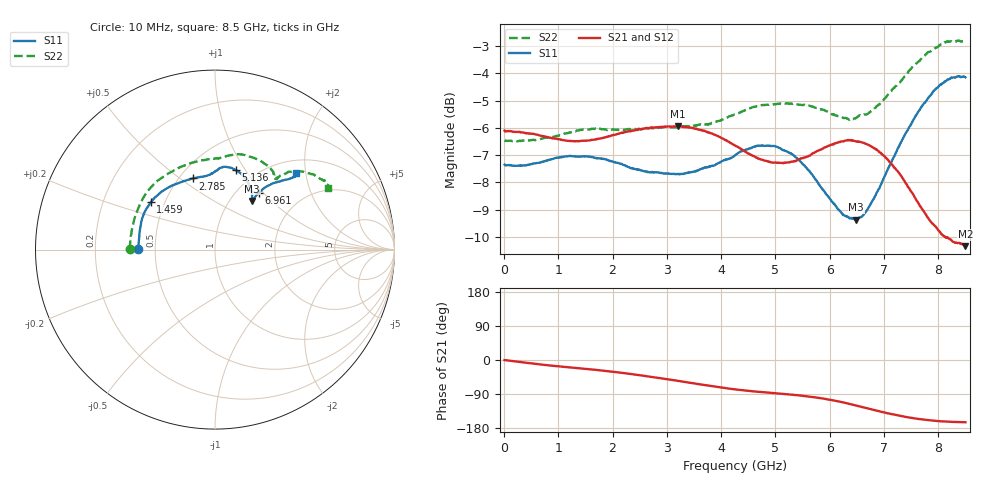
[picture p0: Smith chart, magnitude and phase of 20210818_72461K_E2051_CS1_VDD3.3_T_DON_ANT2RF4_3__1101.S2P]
!Agilent Technologies,E5071C,MY46417908,A.11.23
!Date: Wed Aug 18 14:34:12 2021
!Data & Calibration Information:
!Freq	S11:SOLT2(ON)	S21:SOLT2(ON)	S12:SOLT2(ON)	S22:SOLT2(ON)
!PortZ  Port1:50+j0  Port2:50+j0
!Above PortZ is port z conversion or system Z0 setting when saving the data.
!When reading, reference impedance value at option line is always used.
# Hz S dB R 50
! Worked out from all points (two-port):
!   1601 points, 10 MHz to 8.5 GHz, reference 50 ohm
!   highest |S21| = -5.94 dB at 3.199 GHz (marker M1); lowest = -10.3 dB at 8.5 GHz (marker M2)
!   |S21| within 3 dB of the highest: start of sweep to 7.688 GHz
!   lowest |S11| = -9.4 dB at 6.489 GHz (marker M3), VSWR 2.03, Z = 62.9 + j38.5 ohm
!   |S11| at or under -10 dB: nowhere
!   |S22| runs from -6.5 to -2.8 dB; largest |S21 - S12| = 0.0015
!   S11 on the Smith chart (normalised r, x): 10 MHz: 0.40, +0.00; 1.459 GHz: 0.42, +0.28; 2.785 GHz: 0.58, +0.56; 5.136 GHz: 0.81, +0.91; 6.961 GHz: 1.25, +0.94; 8.5 GHz: 1.28, +1.77
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1e7  -7.35 179.6  -6.10 -0.3  -6.10 -0.3  -6.45 179.6
7.847125e8  -7.20 161.2  -6.33 -13.5  -6.33 -13.5  -6.36 158.7
1.426769e9  -7.05 144.5  -6.48 -22.5  -6.48 -22.4  -6.07 139.2
1.458606e9  -7.04 143.6  -6.47 -22.9  -6.47 -22.8  -6.07 138.3
2.238625e9  -7.39 122.1  -6.15 -35.1  -6.15 -35.2  -6.06 115.6
2.785169e9  -7.63 107.3  -5.98 -46.0  -5.98 -46.1  -6.01 102.9
2.843538e9  -7.64 106.1  -5.97 -47.3  -5.97 -47.3  -6.00 101.6
3.199056e9  -7.69 99.3  -5.94 -55.0  -5.94 -55.0  -5.96 95.5
3.692538e9  -7.45 92.8  -6.10 -66.0  -6.10 -66.0  -5.86 88.6
4.255e9  -7.01 87.8  -6.65 -77.5  -6.64 -77.5  -5.50 81.4
4.700725e9  -6.66 83.2  -7.14 -84.1  -7.13 -84.1  -5.19 74.4
5.135838e9  -6.81 75.2  -7.29 -89.3  -7.29 -89.3  -5.11 65.4
5.671769e9  -7.71 63.1  -6.96 -97.2  -6.98 -97.2  -5.22 55.9
6.138719e9  -8.96 54.7  -6.55 -108.7  -6.56 -108.8  -5.57 51.0
6.488931e9  -9.36 52.7  -6.50 -120.2  -6.50 -120.3  -5.64 48.7
6.679956e9  -9.04 52.7  -6.59 -127.0  -6.59 -127.0  -5.50 49.2
6.961188e9  -8.00 52.2  -6.96 -137.0  -6.96 -137.0  -5.04 48.0
7.088538e9  -7.44 51.8  -7.21 -141.3  -7.23 -141.3  -4.75 47.1
7.544875e9  -5.70 46.8  -8.46 -153.8  -8.46 -153.8  -3.73 42.0
7.926925e9  -4.62 43.0  -9.58 -160.1  -9.57 -160.2  -3.09 35.5
8.139175e9  -4.29 42.2  -10.03 -162.4  -10.01 -162.4  -2.86 32.1
8.5e9  -4.14 43.1  -10.34 -164.3  -10.32 -164.4  -2.88 28.6
